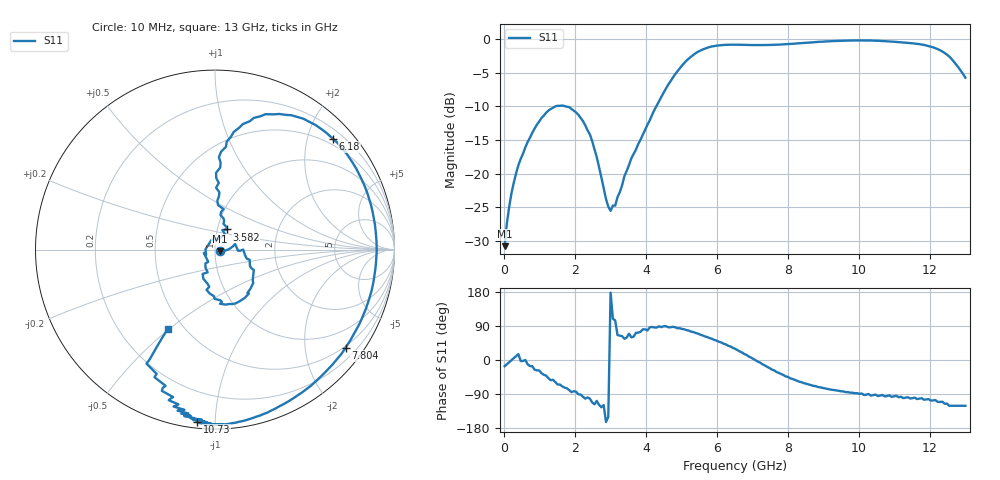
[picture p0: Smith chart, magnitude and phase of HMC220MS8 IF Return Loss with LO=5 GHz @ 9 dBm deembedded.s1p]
!Hittite Microwave Corporation
!12 Elizabeth Drive
!Chelmsford, MA 01824
!Tel: 978-250-3343
!Fax: 978-250-3373
!Device: HMC220MS8, 5-12 GHz, GaAS MMIC SMT Double-Balanced Mixer in 8-lead MSOP package
!Misc: IF Return Loss, LO = 5 GHz @ 9dBm, Room
# MHZ S MA R 50
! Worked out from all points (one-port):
!   201 points, 10 MHz to 13 GHz, reference 50 ohm
!   lowest |S11| = -30.8 dB at 10 MHz (marker M1), VSWR 1.06, Z = 52.9 - j0.869 ohm
!   |S11| at or under -10 dB: start of sweep to 1.444 GHz; 1.727 GHz to 4.286 GHz (2.559 GHz wide, 85.1 % of centre)
!   S11 on the Smith chart (normalised r, x): 10 MHz: 1.06, -0.02; 3.582 GHz: 1.11, +0.25; 6.18 GHz: 0.37, +2.48; 7.804 GHz: 0.46, -2.93; 10.73 GHz: 0.03, -0.90; 13 GHz: 0.41, -0.49
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10  0.029 -16.5
204.85  0.072 -0.3
594.55  0.157 0.1
1049.2  0.259 -34.9
1633.75  0.321 -69.4
2088.4  0.274 -90.5
2413.15  0.196 -101.8
2997.7  0.053 177.7
3257.5  0.073 64.3
3582.25  0.13 59.8
4361.65  0.345 89.0
4881.25  0.576 83.9
5465.8  0.805 69.6
5855.5  0.88 56.0
6180.25  0.902 43.2
6505  0.907 29.7
7089.55  0.901 -0.5
7804  0.91 -36.9
8128.75  0.921 -50.2
8843.2  0.951 -71.3
9752.5  0.975 -86.1
10726.75  0.963 -96.0
10856.65  0.959 -93.4
11246.35  0.943 -100.5
11376.25  0.936 -98.3
12155.65  0.854 -105.8
12545.35  0.741 -121.0
13000  0.516 -120.8
